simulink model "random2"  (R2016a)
settings: Solver=VariableStepDiscrete  StartTime=0.0  StopTime=1e4  RelTol=1e-3
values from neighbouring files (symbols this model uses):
  high = str2double(get_param('random3/Bereichszaehler', 'high'))    [plot_random3.m]
  low = str2double(get_param('random3/Bereichszaehler', 'low'))    [plot_random3.m]
libraries: simulink x5

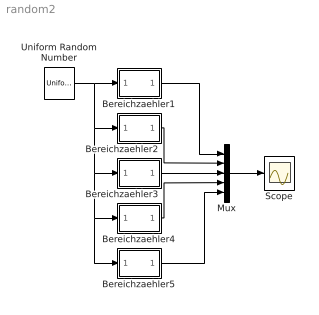
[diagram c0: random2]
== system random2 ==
  Bereichzaehler1 : Subsystem
  Bereichzaehler2 : Subsystem
  Bereichzaehler3 : Subsystem
  Bereichzaehler4 : Subsystem
  Bereichzaehler5 : Subsystem
  Mux : Mux  Inputs=5
  Scope : Scope
  Uniform Random Number : UniformRandomNumber  Minimum=0  SampleTime=1
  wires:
  Uniform Random Number/1 -> Bereichzaehler4/1(In), Bereichzaehler5/1(In), Bereichzaehler3/1(In), Bereichzaehler2/1(In), Bereichzaehler1/1(In)
  Bereichzaehler3/1(Anteil) -> Mux/3
  Bereichzaehler2/1(Anteil) -> Mux/2
  Bereichzaehler1/1(Anteil) -> Mux/1
  Bereichzaehler4/1(Anteil) -> Mux/4
  Bereichzaehler5/1(Anteil) -> Mux/5
  Mux/1 -> Scope/1

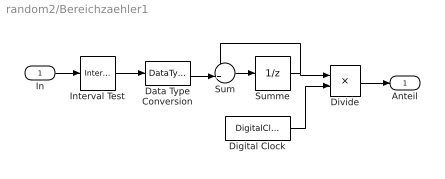
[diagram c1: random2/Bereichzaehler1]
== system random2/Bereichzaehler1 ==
  In : Inport
  Data Type Conversion : DataTypeConversion  OutDataTypeStr=double
  Digital Clock : DigitalClock
  Divide : Product  Inputs=*/
  Interval Test : simulink/Logic and Bit Operations/Interval Test  SystemSampleTime=-1  IntervalClosedRight=on  uplimit=high  IntervalClosedLeft=off  lowlimit=low  LogicOutDataTypeMode=uint8
  Sum : Sum  Inputs=++|
  Summe : UnitDelay  SampleTime=-1
  Anteil : Outport
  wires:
  Sum/1 -> Summe/1
  Summe/1 -> Sum/1, Divide/1
  In/1 -> Interval Test/1
  Divide/1 -> Anteil/1
  Digital Clock/1 -> Divide/2
  Interval Test/1 -> Data Type Conversion/1
  Data Type Conversion/1 -> Sum/2

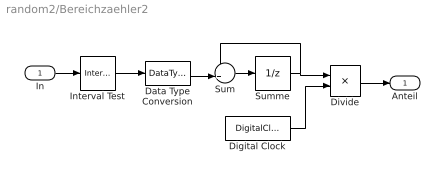
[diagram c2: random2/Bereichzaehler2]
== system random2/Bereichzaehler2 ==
  In : Inport
  Data Type Conversion : DataTypeConversion  OutDataTypeStr=double
  Digital Clock : DigitalClock
  Divide : Product  Inputs=*/
  Interval Test : simulink/Logic and Bit Operations/Interval Test  SystemSampleTime=-1  IntervalClosedRight=on  uplimit=high  IntervalClosedLeft=off  lowlimit=low  LogicOutDataTypeMode=uint8
  Sum : Sum  Inputs=++|
  Summe : UnitDelay  SampleTime=-1
  Anteil : Outport
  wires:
  Sum/1 -> Summe/1
  Summe/1 -> Sum/1, Divide/1
  In/1 -> Interval Test/1
  Divide/1 -> Anteil/1
  Digital Clock/1 -> Divide/2
  Interval Test/1 -> Data Type Conversion/1
  Data Type Conversion/1 -> Sum/2

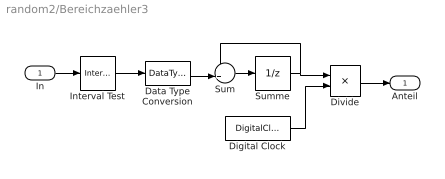
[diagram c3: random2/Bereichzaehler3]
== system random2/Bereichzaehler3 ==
  In : Inport
  Data Type Conversion : DataTypeConversion  OutDataTypeStr=double
  Digital Clock : DigitalClock
  Divide : Product  Inputs=*/
  Interval Test : simulink/Logic and Bit Operations/Interval Test  SystemSampleTime=-1  IntervalClosedRight=on  uplimit=high  IntervalClosedLeft=off  lowlimit=low  LogicOutDataTypeMode=uint8
  Sum : Sum  Inputs=++|
  Summe : UnitDelay  SampleTime=-1
  Anteil : Outport
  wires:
  Sum/1 -> Summe/1
  Summe/1 -> Sum/1, Divide/1
  In/1 -> Interval Test/1
  Divide/1 -> Anteil/1
  Digital Clock/1 -> Divide/2
  Interval Test/1 -> Data Type Conversion/1
  Data Type Conversion/1 -> Sum/2

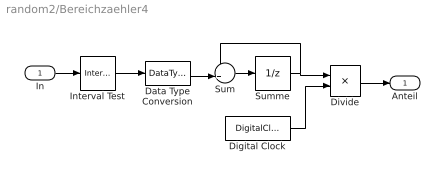
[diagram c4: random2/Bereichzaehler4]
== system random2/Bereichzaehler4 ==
  In : Inport
  Data Type Conversion : DataTypeConversion  OutDataTypeStr=double
  Digital Clock : DigitalClock
  Divide : Product  Inputs=*/
  Interval Test : simulink/Logic and Bit Operations/Interval Test  SystemSampleTime=-1  IntervalClosedRight=on  uplimit=high  IntervalClosedLeft=off  lowlimit=low  LogicOutDataTypeMode=uint8
  Sum : Sum  Inputs=++|
  Summe : UnitDelay  SampleTime=-1
  Anteil : Outport
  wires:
  Sum/1 -> Summe/1
  Summe/1 -> Sum/1, Divide/1
  In/1 -> Interval Test/1
  Divide/1 -> Anteil/1
  Digital Clock/1 -> Divide/2
  Interval Test/1 -> Data Type Conversion/1
  Data Type Conversion/1 -> Sum/2

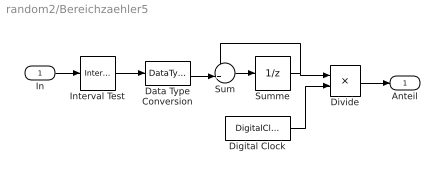
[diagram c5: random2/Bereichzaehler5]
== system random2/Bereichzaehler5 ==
  In : Inport
  Data Type Conversion : DataTypeConversion  OutDataTypeStr=double
  Digital Clock : DigitalClock
  Divide : Product  Inputs=*/
  Interval Test : simulink/Logic and Bit Operations/Interval Test  SystemSampleTime=-1  IntervalClosedRight=on  uplimit=high  IntervalClosedLeft=off  lowlimit=low  LogicOutDataTypeMode=uint8
  Sum : Sum  Inputs=++|
  Summe : UnitDelay  SampleTime=-1
  Anteil : Outport
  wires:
  Sum/1 -> Summe/1
  Summe/1 -> Sum/1, Divide/1
  In/1 -> Interval Test/1
  Divide/1 -> Anteil/1
  Digital Clock/1 -> Divide/2
  Interval Test/1 -> Data Type Conversion/1
  Data Type Conversion/1 -> Sum/2
